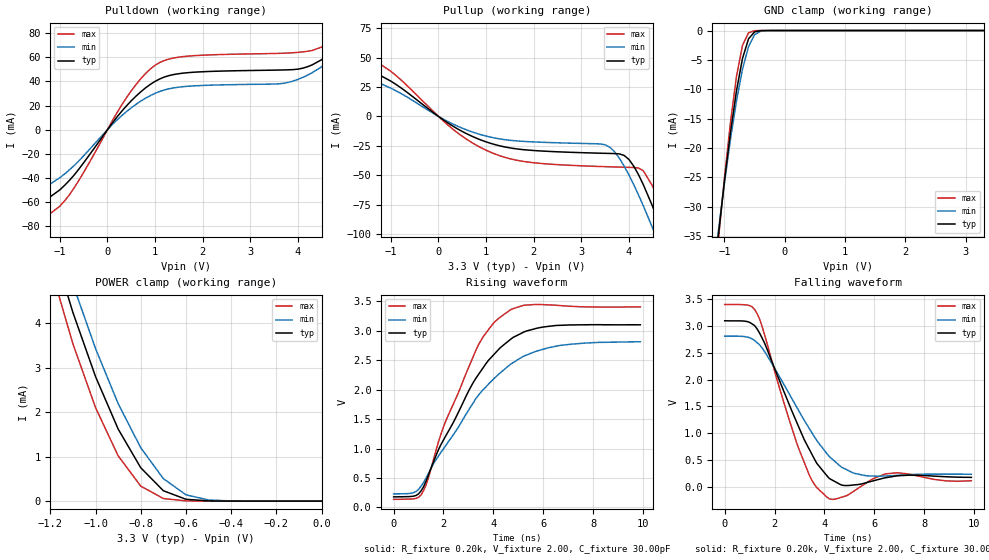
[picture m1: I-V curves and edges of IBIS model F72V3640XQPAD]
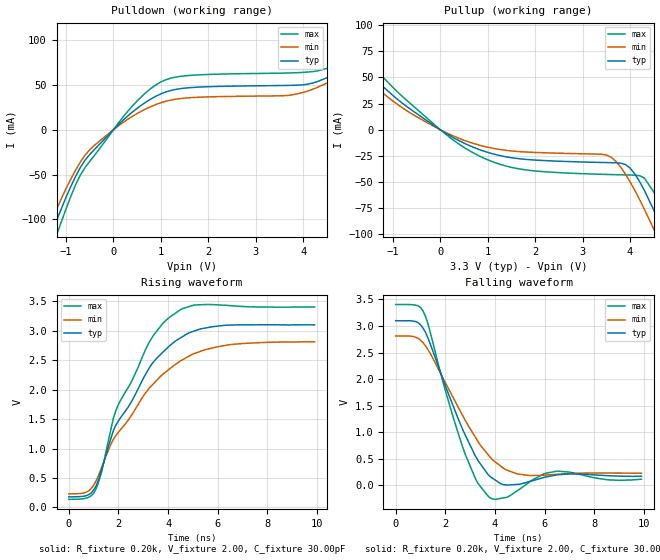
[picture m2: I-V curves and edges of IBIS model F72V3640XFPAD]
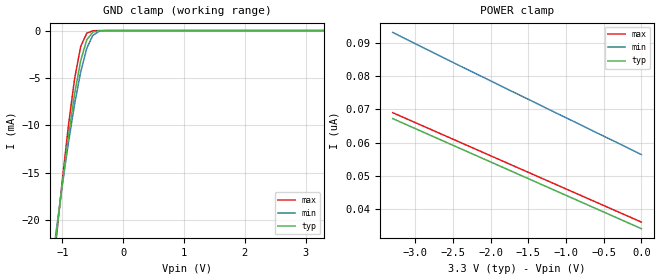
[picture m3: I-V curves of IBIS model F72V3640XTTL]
| IBIS file 72v3640p.ibs created by s2ibis2 version 1.1
| North Carolina State University Electronics Research Laboratory  1995
[IBIS ver]   2.1
[File name]   72v3640p.ibs
[File Rev]   1.0
[Date]   08/30/2001
[Source]   Integrated Device Technology, Inc.
[Notes]   1. Temperatures: typ=25C, min=85C, max=-40C 2. Cemos11.5_3v
   process. 3. Ramp rates based on 50 ohm load.
[Copyright]   Copyright 1999, Integrated Device Technology, Inc.
|   Component idt72v3640x
[Component]   idt72v3640x
[Manufacturer]   Integrated Device Technology
[Package]
| variable   typ   min   max
R_pkg   0.75   0.60   0.90
L_pkg   8.80nH   8.30nH   9.90nH
C_pkg   0.53pF   0.46pF   0.60pF
[Pin]  signal_name   model_name   R_pin   L_pin   C_pin
1   WENL   F72V3640XTTL
2   SENL   F72V3640XTTL
|3   DNC   dummy_model
4   VCC   POWER
|5   DNC   dummy_model
6   IW   F72V3640XTTL
7   D35   F72V3640XTTL
8   D34   F72V3640XTTL
9   D33   F72V3640XTTL
10   D32   F72V3640XTTL
11   VCC   POWER
12   D31   F72V3640XTTL
13   D30   F72V3640XTTL
14   GND   GND
15   D29   F72V3640XTTL
16   D28   F72V3640XTTL
17   D27   F72V3640XTTL
18   D26   F72V3640XTTL
19   D25   F72V3640XTTL
20   D24   F72V3640XTTL
21   D23   F72V3640XTTL
22   GND   GND
23   D22   F72V3640XTTL
24   VCC   POWER
25   D21   F72V3640XTTL
26   D20   F72V3640XTTL
27   D19   F72V3640XTTL
28   D18   F72V3640XTTL
29   GND   GND
30   D17   F72V3640XTTL
31   D16   F72V3640XTTL
32   D15   F72V3640XTTL
33   D14   F72V3640XTTL
34   D13   F72V3640XTTL
35   VCC   POWER
36   D12   F72V3640XTTL
37   GND   GND
38   D11   F72V3640XTTL
39   D10   F72V3640XTTL
40   D9   F72V3640XTTL
41   D8   F72V3640XTTL
42   D7   F72V3640XTTL
43   D6   F72V3640XTTL
44   GND   GND
45   D5   F72V3640XTTL
46   D4   F72V3640XTTL
47   D3   F72V3640XTTL
48   VCC   POWER
49   D2   F72V3640XTTL
50   D1   F72V3640XTTL
51   D0   F72V3640XTTL
52   GND   GND
53   Q0   F72V3640XQPAD
54   Q1   F72V3640XQPAD
55   Q2   F72V3640XQPAD
56   Q3   F72V3640XQPAD
57   Q4   F72V3640XQPAD
58   Q5   F72V3640XQPAD
59   GND   GND
60   Q6   F72V3640XQPAD
61   VCC   POWER
62   Q7   F72V3640XQPAD
63   Q8   F72V3640XQPAD
64   Q9   F72V3640XQPAD
65   Q10   F72V3640XQPAD
66   Q11   F72V3640XQPAD
67   GND   GND
68   Q12   F72V3640XQPAD
69   Q13   F72V3640XQPAD
70   Q14   F72V3640XQPAD
71   Q15   F72V3640XQPAD
72   VCC   POWER
73   VCC   POWER
74   Q16   F72V3640XQPAD
75   Q17   F72V3640XQPAD
76   GND   GND
77   Q18   F72V3640XQPAD
78   Q19   F72V3640XQPAD
79   Q20   F72V3640XQPAD
80   Q21   F72V3640XQPAD
81   Q22   F72V3640XQPAD
82   Q23   F72V3640XQPAD
83   GND   GND
84   GND   GND
85   Q24   F72V3640XQPAD
86   Q25   F72V3640XQPAD
87   VCC   POWER
88   Q26   F72V3640XQPAD
89   Q27   F72V3640XQPAD
90   Q28   F72V3640XQPAD
91   Q29   F72V3640XQPAD
92   Q30   F72V3640XQPAD
93   Q31   F72V3640XQPAD
94   GND   GND
95   GND   GND
96   Q32   F72V3640XQPAD
97   Q33   F72V3640XQPAD
98   Q34   F72V3640XQPAD
99   Q35   F72V3640XQPAD
100   VCC   POWER
101   VCC   POWER
102   OEL   F72V3640XTTL
103   RTL   F72V3640XTTL
104   RENL   F72V3640XTTL
105   RCLK   F72V3640XTTL
106   GND   GND
107   RM   F72V3640XTTL
108   EFL   F72V3640XFPAD
109   PFM   F72V3640XTTL
110   PAEL   F72V3640XFPAD
111   VCC   POWER
112   BM   F72V3640XTTL
113   IP   F72V3640XTTL
114   BEL   F72V3640XTTL
115   FS1   F72V3640XTTL
116   GND   GND
117   HFL   F72V3640XFPAD
118   FS0   F72V3640XTTL
119   OW   F72V3640XTTL
120   GND   GND
121   PAFL   F72V3640XFPAD
122   VCC   POWER
123   FFL   F72V3640XFPAD
124   FWFTSI   F72V3640XTTL
125   LDL   F72V3640XTTL
126   MRSL   F72V3640XTTL
127   PRSL   F72V3640XTTL
128   WCLK   F72V3640XTTL
| Models and submodels in the file (3): F72V3640XQPAD (3-state), F72V3640XFPAD (Output), F72V3640XTTL (Input)
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| FIN  FIN   dummy_model
| QIN  QIN   dummy_model
| QOEL QOEL   dummy_model
|   Model F72V3640XQPAD
[Model]   F72V3640XQPAD
Model_type   3-state
Polarity   Non-Inverting
Enable   Active-Low
Vmeas =  1.500V
C_comp   3.00pF   NA   NA
[Temperature Range]   25.00   85.00   -40.00
[Voltage Range]   3.30V   3.00V   3.60V
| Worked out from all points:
|   slope of the pulldown table from 0 to 0.495 V, typ, clamps not added: 20.9 ohm
|   slope of the pullup table from 0 to 0.495 V, typ, clamps not added: 39 ohm
|   GND clamp passes 1 mA (typ) near -0.57 V on its own axis
|   POWER clamp passes 1 mA (typ) near -0.83 V on its own axis
|   rising waveform, R_fixture 0.20k, V_fixture 2.00, C_fixture 30.00pF: 20-80 % time 2.26ns typ, 2.7ns min, 1.81ns max; typ from 0.179 V to 3.1 V
|   falling waveform, R_fixture 0.20k, V_fixture 2.00, C_fixture 30.00pF: 20-80 % time 1.58ns typ, 1.99ns min, 1.27ns max; typ from 3.1 V to 0.172 V
[Pulldown]
| voltage   I(typ)   I(min)   I(max)
-3.3V     -78.1mA    -69.1mA    -88.4mA
-1.9V     -70.5mA    -59.2mA    -83.7mA
-1.5V     -64.03mA   -52.53mA   -78.38mA
-1V       -49.8mA    -39.74mA   -63.32mA
-600mV    -32.63mA   -25.8mA    -41.94mA
400mV     19.75mA    15.01mA    26.5mA
1.1V      42.09mA    31.72mA    55.68mA
3.8V      49.61mA    39.21mA    63.53mA
4.5V      58.01mA    52.1mA     68.44mA
4.9V      71.41mA    65.07mA    81.85mA
5.3V      92.34mA    83.36mA    107mA
6.6V      239mA      203mA      293mA
[Pullup]
| voltage   I(typ)   I(min)   I(max)
-3.3V     63.83mA    53.96mA    75.83mA
-1.5V     40.98mA    32.98mA    51.93mA
300mV     -8.18mA    -6.429mA   -10.76mA
1.1V      -22.96mA   -17.67mA   -30.55mA
1.9V      -28.69mA   -21.5mA    -38.93mA
3.5V      -31.4mA    -24.13mA   -42.74mA
4V        -36.59mA   -49.74mA   -43.32mA
4.3V      -57.78mA   -75.78mA   -46.12mA
4.5V      -76.76mA   -95.06mA   -59.46mA
4.7V      -97.6mA    -115mA     -79.6mA
4.9V      -119mA     -136mA     -102mA
6.6V      -313mA     -320mA     -309mA
[GND_clamp]
| voltage   I(typ)   I(min)   I(max)
-3.3V     -278mA     -262mA     -298mA
-1.1V     -34.79mA   -34.08mA   -35.63mA
-1V       -25.68mA   -25.97mA   -25.14mA
-900mV    -17.4mA    -18.54mA   -15.66mA
-800mV    -10.26mA   -11.98mA   -7.802mA
-700mV    -4.731mA   -6.568mA   -2.51mA
-600mV    -1.413mA   -2.718mA   -390uA
-500mV    -228uA     -719uA     -31.26uA
-400mV    -22.15uA   -115uA     -1.32uA
-300mV    -1.402uA   -12.89uA   -32.97nA
3.3V      34.83nA    488nA      33.01nA
[POWER_clamp]
| voltage   I(typ)   I(min)   I(max)
-3.3V     72.27mA    66.54mA    80.97mA
-1.2V     5.92mA     6.51mA     5.285mA
-1.1V     4.244mA    4.879mA    3.539mA
-1V       2.802mA    3.433mA    2.105mA
-900mV    1.623mA    2.194mA    1.02mA
-800mV    751uA      1.201mA    338uA
-700mV    234uA      506uA      58.4uA
-600mV    41.73uA    142uA      5.351uA
-500mV    4.842uA    25.8uA     348nA
-400mV    454nA      3.649uA    51.06nA
0V        34.83nA    78.19nA    36.01nA
[Ramp]
| variable   typ   min   max
dV/dt_r   0.86/0.74n   0.65/0.97n   1.13/0.58n
dV/dt_f   1.29/0.94n   1.02/1.24n   1.58/0.64n
R_load = 50.00
[Rising Waveform]
R_fixture = 0.20k
V_fixture = 2.00
C_fixture = 30.00pF
R_dut = 0.75
L_dut = 8.10nH
C_dut = 0.53pF
| time   V(typ)   V(min)   V(max)
0s        179mV      229mV      137mV
800ps     191mV      250mV      146mV
1.1ns     281mV      361mV      211mV
1.3ns     446mV      500mV      381mV
2ns       1.146V     996mV      1.368V
3.3ns     2.193V     1.848V     2.668V
4.2ns     2.677V     2.256V     3.205V
5.2ns     2.973V     2.564V     3.43V
6.2ns     3.073V     2.71V      3.439V
9.9ns     3.1V       2.812V     3.404V
[Falling Waveform]
R_fixture = 0.20k
V_fixture = 2.00
C_fixture = 30.00pF
R_dut = 0.75
L_dut = 8.10nH
C_dut = 0.53pF
| time   V(typ)   V(min)   V(max)
0s        3.1V       2.813V     3.405V
1ns       3.071V     2.783V     3.384V
1.3ns     2.949V     2.691V     3.236V
1.8ns     2.45V      2.375V     2.505V
3ns       1.083V     1.394V     676mV
3.5ns     603mV      1.006V     116mV
4.2ns     150mV      560mV      -231mV
5.2ns     30.62mV    247mV      -80.64mV
6.5ns     169mV      199mV      239mV
9.9ns     172mV      230mV      109mV
|   Model F72V3640XFPAD
[Model]   F72V3640XFPAD
Model_type   Output
Polarity   Non-Inverting
Enable   Active-Low
Vmeas =  1.500V
C_comp   3.00pF   NA   NA
[Temperature Range]   25.00   85.00   -40.00
[Voltage Range]   3.30V   3.00V   3.60V
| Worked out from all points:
|   slope of the pulldown table from 0 to 0.495 V, typ, clamps not added: 20.9 ohm
|   slope of the pullup table from 0 to 0.495 V, typ, clamps not added: 39 ohm
|   rising waveform, R_fixture 0.20k, V_fixture 2.00, C_fixture 30.00pF: 20-80 % time 2.1ns typ, 2.51ns min, 1.75ns max; typ from 0.179 V to 3.1 V
|   falling waveform, R_fixture 0.20k, V_fixture 2.00, C_fixture 30.00pF: 20-80 % time 1.49ns typ, 1.82ns min, 1.2ns max; typ from 3.1 V to 0.172 V
[Pulldown]
| voltage   I(typ)   I(min)   I(max)
-3.3V     -2.813A    -331mA     -386mA
-1.5V     -140mA     -123mA     -161mA
-1V       -75.48mA   -65.71mA   -88.46mA
-700mV    -42.28mA   -36.27mA   -50.74mA
-500mV    -27.61mA   -22.34mA   -35.37mA
400mV     19.75mA    15.01mA    26.5mA
1.1V      42.09mA    31.72mA    55.68mA
4V        50.16mA    41.67mA    64.04mA
4.9V      71.41mA    65.07mA    81.85mA
5.3V      92.34mA    83.36mA    107mA
5.7V      123mA      109mA      145mA
6.6V      239mA      203mA      293mA
[Pullup]
| voltage   I(typ)   I(min)   I(max)
-3.3V     136mA      120mA      157mA
-2.5V     97.91mA    85.33mA    115mA
-2.1V     79.57mA    68.81mA    94.27mA
-700mV    21.96mA    17.97mA    27.81mA
900mV     -20.19mA   -15.64mA   -26.76mA
3.5V      -31.4mA    -24.13mA   -42.74mA
4V        -36.59mA   -49.74mA   -43.32mA
4.3V      -57.78mA   -75.78mA   -46.12mA
4.5V      -76.76mA   -95.06mA   -59.46mA
4.7V      -97.6mA    -115mA     -79.6mA
4.9V      -119mA     -136mA     -102mA
6.6V      -313mA     -320mA     -309mA
[Ramp]
| variable   typ   min   max
dV/dt_r   0.86/0.44n   0.65/0.52n   1.13/0.39n
dV/dt_f   1.29/0.69n   1.02/0.88n   1.58/0.51n
R_load = 50.00
[Rising Waveform]
R_fixture = 0.20k
V_fixture = 2.00
C_fixture = 30.00pF
R_dut = 0.75
L_dut = 8.10nH
C_dut = 0.53pF
| time   V(typ)   V(min)   V(max)
0s        179mV      229mV      137mV
1ns       297mV      375mV      239mV
1.3ns     609mV      657mV      565mV
1.8ns     1.31V      1.159V     1.524V
2ns       1.471V     1.278V     1.749V
3.3ns     2.41V      2.052V     2.849V
4.1ns     2.76V      2.365V     3.242V
5ns       2.988V     2.606V     3.431V
6ns       3.079V     2.729V     3.44V
9.9ns     3.1V       2.813V     3.404V
[Falling Waveform]
R_fixture = 0.20k
V_fixture = 2.00
C_fixture = 30.00pF
R_dut = 0.75
L_dut = 8.10nH
C_dut = 0.53pF
| time   V(typ)   V(min)   V(max)
0s        3.1V       2.813V     3.405V
800ps     3.084V     2.79V      3.394V
1.1ns     2.961V     2.688V     3.286V
2.8ns     948mV      1.226V     586mV
3.3ns     480mV      839mV      46.94mV
3.8ns     167mV      536mV      -235mV
4.3ns     19.09mV    338mV      -238mV
4.9ns     19.4mV     215mV      -100mV
6.5ns     199mV      209mV      268mV
9.9ns     172mV      230mV      117mV
|   Model F72V3640XTTL
[Model]   F72V3640XTTL
Model_type   Input
Vinl =  0.000V
Vinh =  3.000V
Vmeas =  1.500V
C_comp   3.00pF   NA   NA
[Temperature Range]   25.00   85.00   -40.00
[Voltage Range]   3.30V   3.00V   3.60V
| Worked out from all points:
|   GND clamp passes 1 mA (typ) near -0.60 V on its own axis
[GND_clamp]
| voltage   I(typ)   I(min)   I(max)
-3.3V     -163mA     -152mA     -175mA
-1.2V     -27.14mA   -26.04mA   -28.44mA
-1.1V     -21.44mA   -20.99mA   -21.88mA
-1V       -16.05mA   -16.21mA   -15.65mA
-900mV    -11.07mA   -11.76mA   -9.94mA
-800mV    -6.681mA   -7.76mA    -5.083mA
-700mV    -3.176mA   -4.372mA   -1.687mA
-600mV    -978uA     -1.868mA   -273uA
-500mV    -164uA     -509uA     -22.75uA
-400mV    -16.27uA   -84.16uA   -951nA
-300mV    -1.023uA   -9.558uA   -24.55nA
3.3V      34.02nA    59.73nA    33.01nA
[POWER_clamp]
| voltage   I(typ)   I(min)   I(max)
-3.3V     67.23nA    93.23nA    69.01nA
-2.9V     63.2nA     88.67nA    65.01nA
-2.3V     57.16nA    81.94nA    59.01nA
0V        34.02nA    56.39nA    36.01nA
